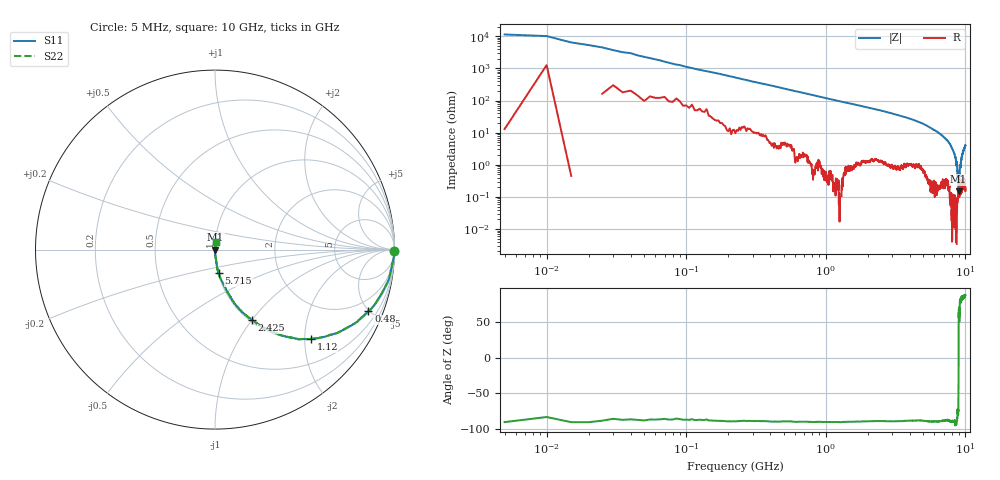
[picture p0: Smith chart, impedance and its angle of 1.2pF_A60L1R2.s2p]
! Amotech Co.,Ltd.
! http://www.amotech.co.kr/
! Part Number: A60L1R2
! These Parameters are Measured in Series Mode Connection
! Operation Temp=25[degC], DC Bias Voltage=0[V]
! Freq. Start=5[MHz] Stop=10[GHz], 2000[Steps]
! Date: Monday, July 14, 2020, 09:45:31
# GHZ S RI R 50.000000
!Freq.(Hz) S11(Real) S11(Imag) S21(Real) S21(Imag) S12(Real) S12(Imag) S22(Real) S22(Imag)
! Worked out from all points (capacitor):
!   2000 points, 5 MHz to 10 GHz, reference 50 ohm
!   read as one part in series: C = 1.41 pF near 55 MHz
!   lowest |Z| = 148 mohm at 8.94 GHz (marker M1)
!   series resonance near 8.935 GHz, so ESL is about 220 pH
!   S11 on the Smith chart (normalised r, x): 5 MHz: open; 480 MHz: 1.10, -4.95; 1.12 GHz: 1.01, -2.14; 2.425 GHz: 1.02, -1.00; 5.715 GHz: 1.01, -0.27; 10 GHz: 1.00, +0.08
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0.005  0.9999 -0.00878  8.72e-05 0.00878  8.72e-05 0.00878  0.9999 -0.00878
0.08  0.9905 -0.07  0.00952 0.07  0.00952 0.07  0.9905 -0.07
0.145  0.9794 -0.1224  0.0206 0.1224  0.0206 0.1224  0.9794 -0.1224
0.285  0.9374 -0.2264  0.0626 0.2264  0.0626 0.2264  0.9374 -0.2264
0.48  0.8549 -0.3425  0.1451 0.3425  0.1451 0.3425  0.8549 -0.3425
1.12  0.5335 -0.4974  0.4665 0.4974  0.4665 0.4974  0.5335 -0.4974
1.675  0.3442 -0.4676  0.6558 0.4676  0.6558 0.4676  0.3442 -0.4676
2.425  0.2067 -0.3929  0.7933 0.3929  0.7933 0.3929  0.2067 -0.3929
3.34  0.1105 -0.3028  0.8895 0.3028  0.8895 0.3028  0.1105 -0.3028
5.005  0.0388 -0.1778  0.9612 0.1778  0.9612 0.1778  0.0388 -0.1778
5.715  0.0204 -0.1308  0.9796 0.1308  0.9796 0.1308  0.0204 -0.1308
6.67  0.00986 -0.0863  0.9901 0.0863  0.9901 0.0863  0.00986 -0.0863
7.56  0.00473 -0.0521  0.9953 0.0521  0.9953 0.0521  0.00473 -0.0521
8.335  0.000937 -0.0221  0.9991 0.0221  0.9991 0.0221  0.000937 -0.0221
8.7  0.000419 -0.012  0.9996 0.012  0.9996 0.012  0.000419 -0.012
8.79  0.000921 -0.0028  0.9991 0.0028  0.9991 0.0028  0.000921 -0.0028
8.865  0.00104 -0.00544  0.999 0.00544  0.999 0.00544  0.00104 -0.00544
8.94  0.00144 0.000327  0.9986 -0.000327  0.9986 -0.000327  0.00144 0.000327
9.035  0.00117 0.00206  0.9988 -0.00206  0.9988 -0.00206  0.00117 0.00206
9.155  0.00216 0.00833  0.9978 -0.00833  0.9978 -0.00833  0.00216 0.00833
9.455  0.0027 0.0189  0.9973 -0.0189  0.9973 -0.0189  0.0027 0.0189
10  0.00333 0.0401  0.9967 -0.0401  0.9967 -0.0401  0.00333 0.0401
